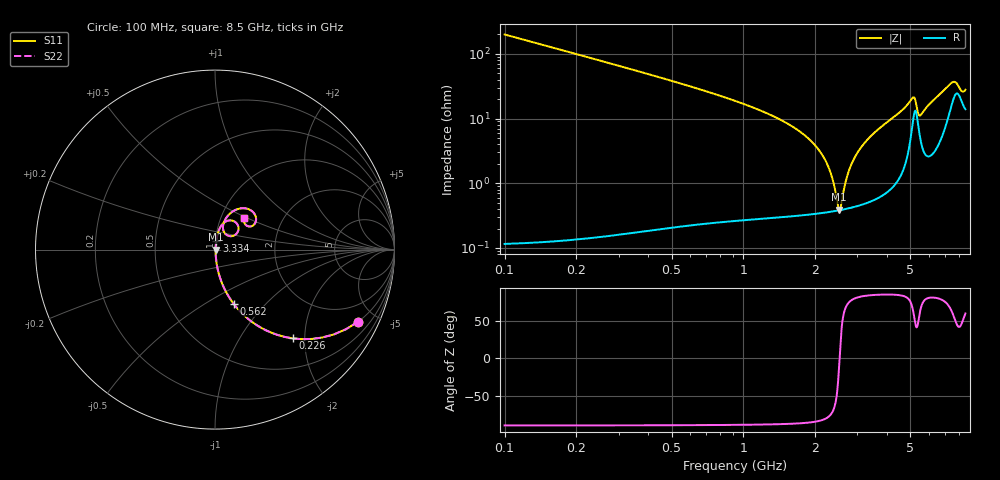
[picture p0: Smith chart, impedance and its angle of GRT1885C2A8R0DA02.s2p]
!Murata Part Number: GRT1885C2A8R0DA02
!These Parameters are Measured in Series Mode Connection
!Data Generated on Jun 19, 2026
!  o--ll--o
!Port1  Port2
!  o------o
!Operation Temp=25[degC], DC Bias Voltage=0[V]
!Freq. Start=100[MHz] Stop=9[GHz] 401[Steps]
# Hz S RI R 50
!Freq.(Hz) S11(Real) S11(Imag) S21(Real) S21(Imag) S12(Real) S12(Imag) S22(Real) S22(Imag)
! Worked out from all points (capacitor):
!   401 points, 100 MHz to 8.5 GHz, reference 50 ohm
!   read as one part in series: C = 8 pF near 142 MHz
!   lowest |Z| = 389 mohm at 2.515 GHz (marker M1)
!   series resonance near 2.526 GHz, so ESL is about 500 pH
!   S11 on the Smith chart (normalised r, x): 100 MHz: 1.00, -3.97; 226 MHz: 1.00, -1.75; 562 MHz: 1.00, -0.67; 3.334 GHz: 1.01, +0.10; 8.5 GHz: 1.28, +0.48
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1e8  0.7976 -0.4015  0.2024 0.4015  0.2024 0.4015  0.7976 -0.4015
2.26e8  0.4325 -0.4946  0.5675 0.4946  0.5675 0.4946  0.4325 -0.4946
3.73e8  0.2145 -0.4088  0.7855 0.4088  0.7855 0.4088  0.2145 -0.4088
5.62e8  0.1032 -0.301  0.8968 0.301  0.8968 0.301  0.1032 -0.301
1.507e9  0.0103 -0.0849  0.9897 0.0849  0.9897 0.0849  0.0103 -0.0849
1.906e9  0.00537 -0.0456  0.9946 0.0456  0.9946 0.0456  0.00537 -0.0456
2.179e9  0.00407 -0.0239  0.9959 0.0239  0.9959 0.0239  0.00407 -0.0239
2.347e9  0.00378 -0.0119  0.9962 0.0119  0.9962 0.0119  0.00378 -0.0119
2.515e9  0.0038 -0.000715  0.9962 0.000715  0.9962 0.000715  0.0038 -0.000715
2.557e9  0.00385 0.002  0.9961 -0.002  0.9961 -0.002  0.00385 0.002
2.725e9  0.0042 0.0125  0.9958 -0.0125  0.9958 -0.0125  0.0042 0.0125
2.914e9  0.00486 0.0239  0.9951 -0.0239  0.9951 -0.0239  0.00486 0.0239
3.334e9  0.00734 0.0479  0.9927 -0.0479  0.9927 -0.0479  0.00734 0.0479
4.3e9  0.0205 0.1046  0.9795 -0.1046  0.9795 -0.1046  0.0205 0.1046
5.119e9  0.1076 0.1569  0.8924 -0.1569  0.8924 -0.1569  0.1076 0.1569
5.224e9  0.1312 0.1171  0.8688 -0.1171  0.8688 -0.1171  0.1312 0.1171
5.434e9  0.068 0.0799  0.932 -0.0799  0.932 -0.0799  0.068 0.0799
5.707e9  0.0442 0.1204  0.9558 -0.1204  0.9558 -0.1204  0.0442 0.1204
7.114e9  0.143 0.2298  0.857 -0.2298  0.857 -0.2298  0.143 0.2298
7.723e9  0.229 0.1736  0.771 -0.1736  0.771 -0.1736  0.229 0.1736
8.185e9  0.1783 0.1327  0.8217 -0.1327  0.8217 -0.1327  0.1783 0.1327
8.5e9  0.1595 0.1772  0.8405 -0.1772  0.8405 -0.1772  0.1595 0.1772
